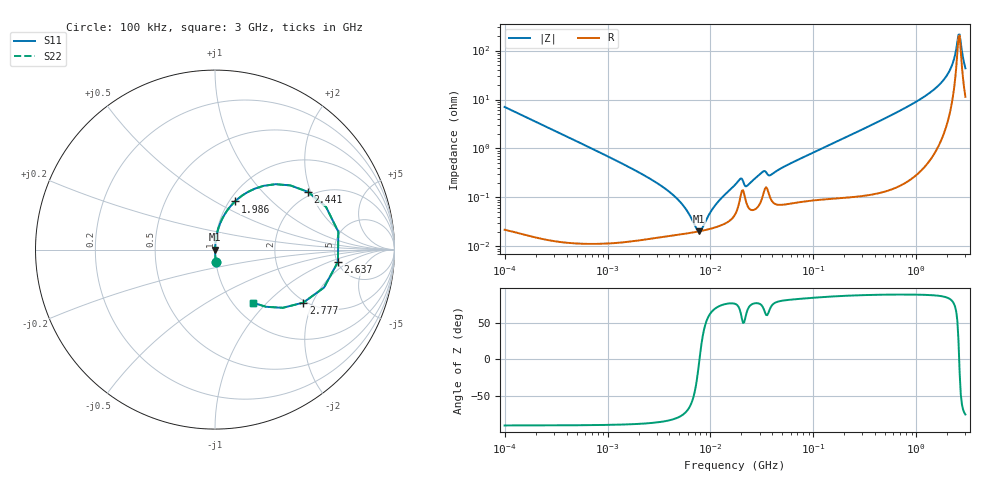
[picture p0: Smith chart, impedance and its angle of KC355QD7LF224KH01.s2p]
!Murata Part Number: KC355QD7LF224KH01
!These Parameters are Measured in Series Mode Connection
!Data Generated on Mar 13, 2026
!  o--ll--o
!Port1  Port2
!  o------o
!Operation Temp=25[degC], DC Bias Voltage=0[V]
!Freq. Start=100[kHz] Stop=3[GHz] 401[Steps]
# Hz S RI R 50
!Freq.(Hz) S11(Real) S11(Imag) S21(Real) S21(Imag) S12(Real) S12(Imag) S22(Real) S22(Imag)
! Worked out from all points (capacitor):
!   401 points, 100 kHz to 3 GHz, reference 50 ohm
!   read as one part in series: C = 225 nF near 105.3 kHz
!   lowest |Z| = 20.3 mohm at 7.791 MHz (marker M1)
!   series resonance near 7.822 MHz, so ESL is about 1.8 nH
!   S11 on the Smith chart (normalised r, x): 100 kHz: 1.00, -0.14; 1.986 GHz: 1.06, +0.62; 2.441 GHz: 1.87, +1.92; 2.637 GHz: 5.06, -1.31; 2.777 GHz: 1.94, -1.71; 3 GHz: 1.23, -0.84
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100000  0.00518 -0.0702  0.9948 0.0702  0.9948 0.0702  0.00518 -0.0702
562235  0.000269 -0.0125  0.9997 0.0125  0.9997 0.0125  0.000269 -0.0125
3161081  0.000155 -0.00185  0.9998 0.00185  0.9998 0.00185  0.000155 -0.00185
5158208  0.000177 -0.000762  0.9998 0.000762  0.9998 0.000762  0.000177 -0.000762
7399428  0.000199 -9.87e-05  0.9998 9.87e-05  0.9998 9.87e-05  0.000199 -9.87e-05
7790830  0.000203 -7e-06  0.9998 7e-06  0.9998 7e-06  0.000203 -7e-06
1.117591e7  0.000245 0.000656  0.9998 -0.000656  0.9998 -0.000656  0.000245 0.000656
1.77727e7  0.000498 0.00185  0.9995 -0.00185  0.9995 -0.00185  0.000498 0.00185
1.970265e7  0.00111 0.00217  0.9989 -0.00217  0.9989 -0.00217  0.00111 0.00217
2.299754e7  0.000664 0.00164  0.9993 -0.00164  0.9993 -0.00164  0.000664 0.00164
3.215051e7  0.00106 0.00316  0.9989 -0.00316  0.9989 -0.00316  0.00106 0.00316
3.850681e7  0.000942 0.00271  0.9991 -0.00271  0.9991 -0.00271  0.000942 0.00271
9.738194e7  0.000926 0.00798  0.9991 -0.00798  0.9991 -0.00798  0.000926 0.00798
5.475153e8  0.00349 0.0456  0.9965 -0.0456  0.9965 -0.0456  0.00349 0.0456
1.281618e9  0.0204 0.1234  0.9796 -0.1234  0.9796 -0.1234  0.0204 0.1234
1.986261e9  0.1115 0.2683  0.8885 -0.2683  0.8885 -0.2683  0.1115 0.2683
2.201951e9  0.2216 0.3395  0.7784 -0.3395  0.7784 -0.3395  0.2216 0.3395
2.318426e9  0.3367 0.3644  0.6633 -0.3644  0.6633 -0.3644  0.3367 0.3644
2.441062e9  0.5183 0.3215  0.4817 -0.3215  0.4817 -0.3215  0.5183 0.3215
2.637286e9  0.685 -0.0683  0.315 0.0683  0.315 0.0683  0.685 -0.0683
2.776789e9  0.4916 -0.2955  0.5084 0.2955  0.5084 0.2955  0.4916 -0.2955
3e9  0.2136 -0.2965  0.7864 0.2965  0.7864 0.2965  0.2136 -0.2965
